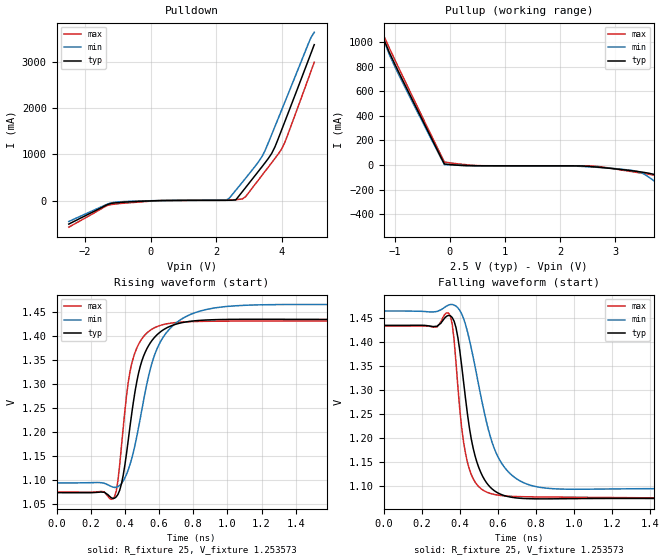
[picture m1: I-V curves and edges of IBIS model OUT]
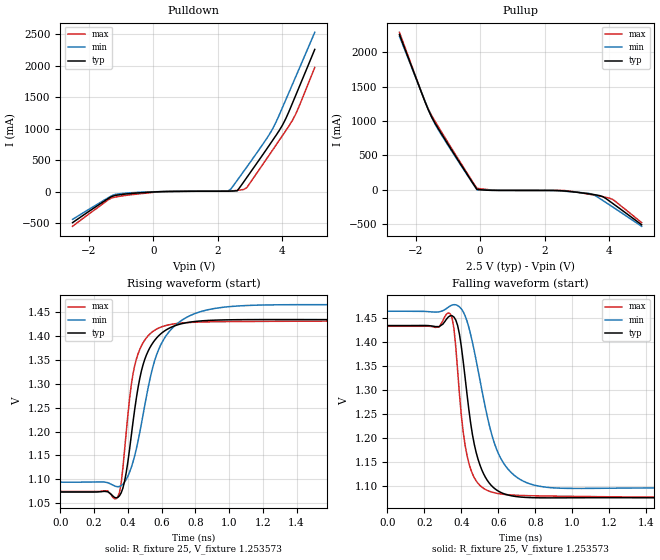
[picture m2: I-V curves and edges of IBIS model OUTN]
|   IBIS File of SG2520VHN D
|   LVDS, Vcc=2.5V, Io=7mA, fo<=212.5MHz
[IBIS Ver]   3.2
[File Name]   sg2520vhn_7m_25v.ibs
[File Rev]   1.0
[Date]   Sep. 23, 2020
[Source]
Fairchild Ensigna Lab's Method
[Notes]
Created by Minoru Kozaki
[Disclaimer]
Seiko Epson Corporation makes no warranty with respect to the
information contained herein.
[Copyright]
Copyright(C) 2020, Seiko Epson Corporation. All rights reserved.
|   Component
[Component]   SG2520VHN
[Manufacturer]  Seiko Epson Corporation
[Package]
R_pkg   17.7m   NA   NA
L_pkg   235p   NA   NA
C_pkg   208f   NA   NA
[Pin]   signal_name   model_name   R_pin   L_pin   C_pin
1   OE/ST   NC
2   NC   NC
3   GND   GND
4   OUT   OUT   17.7m   235p   208f
5   OUTN   OUTN   10.4m   129p   221f
6   VCC   POWER
[Diff Pin] inv_pin  vdiff  tdelay_typ
4   5   0   0
| Models and submodels in the file (2): OUT (Output), OUTN (Output)
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|   Model OUT
[Model]   OUT
Model_type   Output
Polarity   Non-Inverting
Vref = 1.25
Vmeas = 1.25
Rref = 25
Cref = 0
C_comp   4.5p   4.5p   4.5p
[Temperature Range]   25   105   -40
[Voltage Range]   2.5   2.25   2.75
[Pullup Reference]   2.5   2.25   2.75
[Pulldown Reference]   0   0   0
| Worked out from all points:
|   slope of the pulldown table from 0 to 0.375 V, typ, clamps not added: 51.2 ohm
|   slope of the pullup table from 0 to 0.375 V, typ, clamps not added: 39.1 ohm
|   falling waveform, R_fixture 25, V_fixture 1.253573: 20-80 % time 88.2ps typ, 134ps min, 64ps max; typ from 1.43 V to 1.07 V
|   rising waveform, R_fixture 25, V_fixture 1.253573: 20-80 % time 108ps typ, 155ps min, 81.3ps max; typ from 1.07 V to 1.43 V
[Pullup]
-2.5V     3.365A     3.267A     3.476A
-1.3V     1.162A     1.171A     1.174A
-1.2V     1.022A     1.017A     1.051A
-1V       820.3mA    799.7mA    856.2mA
-100mV    7.598mA    2.472mA    23.83mA
500mV     -6.849mA   -6.81mA    -5.288mA
2.6V      -15.05mA   -17.28mA   -9.299mA
3.4V      -52.8mA    -52.3mA    -61.43mA
3.5V      -59.34mA   -67.75mA   -68.49mA
3.8V      -95.8mA    -159mA     -91.03mA
4.1V      -202.9mA   -253.8mA   -134.6mA
5V        -522.6mA   -540.8mA   -496.3mA
[Pulldown]
-2.5V     -505mA     -449.2mA   -571.4mA
-1.2V     -57.92mA   -44.8mA    -82.69mA
300mV     2.554mA    2.651mA    2.312mA
2.4V      9.755mA    50.87mA    12.27mA
2.6V      15.48mA    222.4mA    22.43mA
2.9V      281.3mA    483.4mA    84.29mA
3.4V      730.3mA    949.7mA    544.4mA
3.7V      1.022A     1.429A     820.4mA
4V        1.522A     1.952A     1.112A
4.1V      1.705A     2.126A     1.256A
4.8V      2.997A     3.356A     2.599A
5V        3.37A      3.637A     2.991A
[Falling Waveform]
R_fixture = 25
V_fixture = 1.253573
V_fixture_min = 1.278673
V_fixture_max = 1.253493
0s        1.434V     1.464V     1.433V
350ps     1.454V     1.477V     1.454V
370ps     1.443V     1.476V     1.403V
390ps     1.408V     1.47V      1.306V
440ps     1.25V      1.421V     1.15V
490ps     1.15V      1.329V     1.103V
580ps     1.091V     1.18V      1.083V
690ps     1.076V     1.118V     1.079V
880ps     1.074V     1.095V     1.078V
4ns       1.073V     1.094V     1.074V
[Rising Waveform]
R_fixture = 25
V_fixture = 1.253573
V_fixture_min = 1.278673
V_fixture_max = 1.253493
0s        1.073V     1.093V     1.074V
340ps     1.061V     1.084V     1.065V
390ps     1.109V     1.097V     1.207V
420ps     1.183V     1.121V     1.304V
450ps     1.263V     1.158V     1.356V
510ps     1.359V     1.267V     1.4V
620ps     1.412V     1.396V     1.424V
780ps     1.431V     1.445V     1.43V
1.05ns    1.435V     1.464V     1.431V
4ns       1.434V     1.464V     1.433V
[Ramp]
R_load = 50
dV/dt_r   0.21699/107.68p   0.22409/156.15p   0.21569/81.46p
dV/dt_f   0.21699/88.06p   0.22409/135.82p   0.21569/63.77p
|   Model OUTN
[Model]   OUTN
Model_type   Output
Polarity   Inverting
Vref = 1.25
Vmeas = 1.25
Rref = 25
Cref = 0
C_comp   4.5p   4.5p   4.5p
[Temperature Range]   25   105   -40
[Voltage Range]   2.5   2.25   2.75
[Pullup Reference]   2.5   2.25   2.75
[Pulldown Reference]   0   0   0
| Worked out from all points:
|   slope of the pulldown table from 0 to 0.375 V, typ, clamps not added: 51.5 ohm
|   slope of the pullup table from 0 to 0.375 V, typ, clamps not added: 39.2 ohm
|   falling waveform, R_fixture 25, V_fixture 1.253573: 20-80 % time 89.5ps typ, 134ps min, 66ps max; typ from 1.43 V to 1.07 V
|   rising waveform, R_fixture 25, V_fixture 1.253573: 20-80 % time 108ps typ, 155ps min, 82.4ps max; typ from 1.07 V to 1.43 V
[Pullup]
-2.5V     2.257A     2.231A     2.289A
-1.8V     1.393A     1.397A     1.397A
-1.6V     1.156A     1.161A     1.168A
-1.5V     1.056A     1.053A     1.078A
-1.3V     892.4mA    876.9mA    920.6mA
-100mV    7.54mA     2.456mA    23.61mA
500mV     -6.848mA   -6.802mA   -5.294mA
2.6V      -15.1mA    -19.41mA   -9.302mA
3.4V      -58.89mA   -54.04mA   -64.99mA
3.8V      -98.34mA   -154.5mA   -98.92mA
4.1V      -194.9mA   -246.8mA   -137.4mA
5V        -506.7mA   -528.5mA   -476mA
[Pulldown]
-2.5V     -490.4mA   -438.3mA   -548.5mA
-1.4V     -109.1mA   -96.1mA    -129.2mA
-1.2V     -61.6mA    -45.6mA    -87.12mA
300mV     2.533mA    2.627mA    2.291mA
2.3V      8.807mA    8.708mA    9.763mA
2.4V      9.711mA    41.61mA    12.21mA
2.6V      15.38mA    182.2mA    22.25mA
2.9V      229.3mA    395.6mA    67.85mA
3.6V      744mA      914.3mA    590.5mA
4V        1.057A     1.336A     891.5mA
4.4V      1.517A     1.813A     1.222A
5V        2.259A     2.53A      1.972A
[Falling Waveform]
R_fixture = 25
V_fixture = 1.253573
V_fixture_min = 1.278673
V_fixture_max = 1.253493
0s        1.434V     1.464V     1.433V
340ps     1.454V     1.475V     1.459V
360ps     1.452V     1.478V     1.428V
390ps     1.416V     1.473V     1.291V
440ps     1.261V     1.431V     1.149V
490ps     1.156V     1.342V     1.106V
580ps     1.095V     1.188V     1.086V
700ps     1.078V     1.118V     1.081V
900ps     1.075V     1.096V     1.079V
4ns       1.074V     1.094V     1.075V
[Rising Waveform]
R_fixture = 25
V_fixture = 1.253573
V_fixture_min = 1.278673
V_fixture_max = 1.253493
0s        1.073V     1.094V     1.075V
340ps     1.062V     1.085V     1.063V
360ps     1.072V     1.087V     1.092V
390ps     1.114V     1.1V       1.198V
420ps     1.191V     1.125V     1.298V
450ps     1.27V      1.164V     1.351V
510ps     1.361V     1.274V     1.396V
630ps     1.414V     1.402V     1.423V
1.1ns     1.434V     1.464V     1.431V
4ns       1.434V     1.464V     1.432V
[Ramp]
R_load = 50
dV/dt_r   0.21497/106.99p   0.21814/150.08p   0.21368/81.55p
dV/dt_f   0.21497/88.72p   0.21814/131.58p   0.21368/65.27p
